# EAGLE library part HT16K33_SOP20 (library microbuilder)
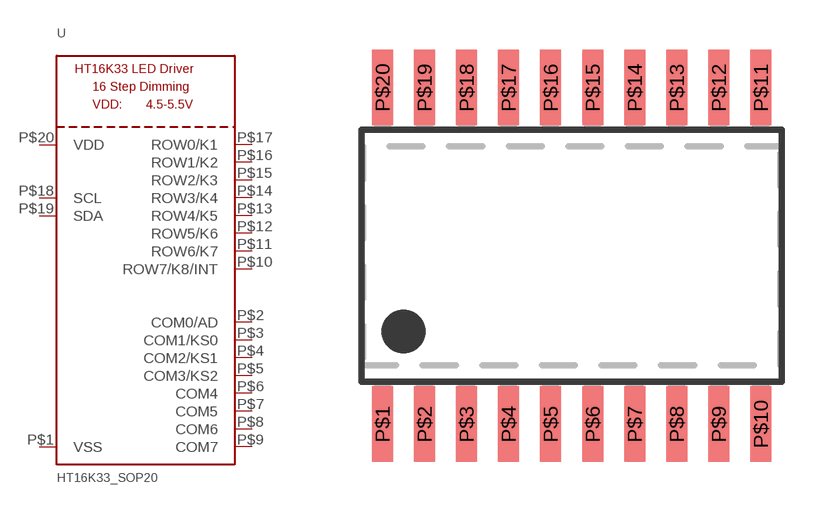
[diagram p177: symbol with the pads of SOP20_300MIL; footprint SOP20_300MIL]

Designator prefix U

## HT16K33_SOP20  [SOP20_300MIL]
P$1  VSS
P$2  COM0/AD
P$3  COM1/KS0
P$4  COM2/KS1
P$5  COM3/KS2
P$6  COM4
P$7  COM5
P$8  COM6
P$9  COM7
P$10  ROW7/K8/INT
P$11  ROW6/K7
P$12  ROW5/K6
P$13  ROW4/K5
P$14  ROW3/K4
P$15  ROW2/K3
P$16  ROW1/K2
P$17  ROW0/K1
P$18  SCL
P$19  SDA
P$20  VDD

## Footprint SOP20_300MIL (pad centres in mm)
smd 0.635 x 2.286: P$1 -5.715,-5.08; P$2 -4.445,-5.08; P$3 -3.175,-5.08; P$4 -1.905,-5.08; P$5 -0.635,-5.08; P$6 0.635,-5.08; P$7 1.905,-5.08; P$8 3.175,-5.08; P$9 4.445,-5.08; P$10 5.715,-5.08; P$11 5.715,5.08; P$12 4.445,5.08; P$13 3.175,5.08; P$14 1.905,5.08; P$15 0.635,5.08; P$16 -0.635,5.08; P$17 -1.905,5.08; P$18 -3.175,5.08; P$19 -4.445,5.08; P$20 -5.715,5.08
